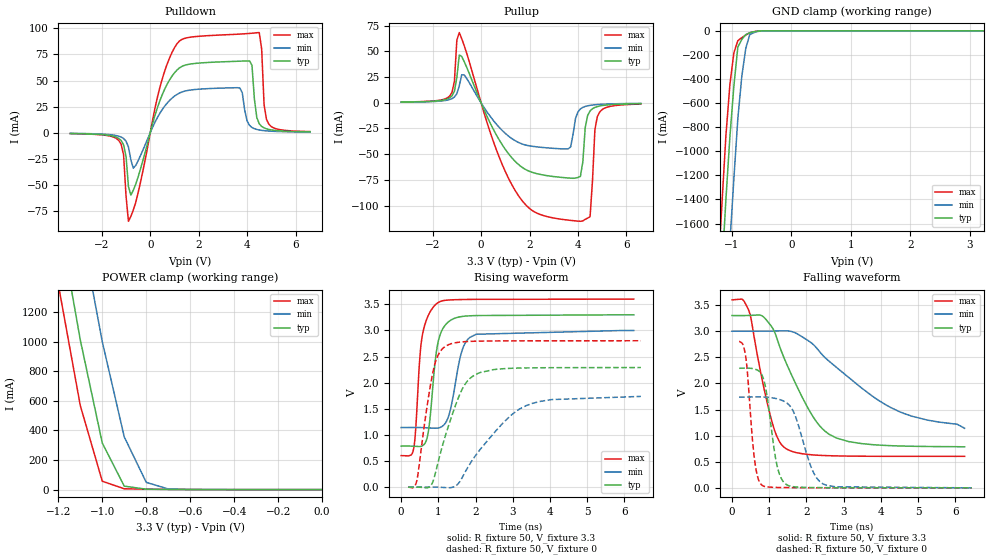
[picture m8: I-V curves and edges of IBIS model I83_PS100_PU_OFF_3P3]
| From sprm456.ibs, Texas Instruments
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|   Model Cell I83_PS100_PU_OFF_3P3
|IDG09_OUI83I83_PS100_PU_OFF_3P3
[Model]   I83_PS100_PU_OFF_3P3
Model_type   I/O
Polarity   Non-Inverting
Enable   Active-Low
Vinl =  0.8V
Vinh =  2V
Cref =  15pF
Rref =  100.00M
Vref =  0V
Vmeas =  1.65
C_comp   5.307p   5.123p   6.171p
[Model Spec]
Vinl   0.8V   0.8V   0.8V
Vinh   2V   2V   2V
[Temperature Range]   25   125   -40
[Voltage Range]   3.3   3   3.6
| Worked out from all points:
|   slope of the pulldown table from 0 to 0.495 V, typ, clamps not added: 13.6 ohm
|   slope of the pullup table from 0 to 0.495 V, typ, clamps not added: 19.6 ohm
|   GND clamp passes 1 mA (typ) near -0.52 V on its own axis
|   POWER clamp passes 1 mA (typ) near -0.67 V on its own axis
|   rising waveform, R_fixture 50, V_fixture 3.3: 20-80 % time 228ps typ, 309ps min, 198ps max; typ from 0.785 V to 3.3 V
|   rising waveform, R_fixture 50, V_fixture 0: 20-80 % time 625ps typ, 1.21ns min, 357ps max; typ from 0 V to 2.29 V
|   falling waveform, R_fixture 50, V_fixture 3.3: 20-80 % time 1.01ns typ, 2.01ns min, 530ps max; typ from 3.3 V to 0.785 V
|   falling waveform, R_fixture 50, V_fixture 0: 20-80 % time 276ps typ, 463ps min, 192ps max; typ from 2.29 V to 0 V
| Nom Voltages:
|   VDD=1.1, VDDS=3.3, VSS=0, VSSS=0
| Min Voltages:
|   VDD=1, VDDS=3, VSS=0, VSSS=0
| Max Voltages:
|   VDD=1.2, VDDS=3.6, VSS=0, VSSS=0
[POWER_clamp]
|   voltage   I(typ)   I(min)   I(max)
-3.3V     22.22A     22.93A     21.83A
-1.2V     1.856A     2.664A     1.387A
-1.167V   1.575A     2.376A     1.114A
-1.133V   1.294A     2.087A     841.3mA
-1.1V     1.013A     1.799A     568.3mA
-1.067V   780mA      1.533A     397.8mA
-1.033V   547.6mA    1.267A     227.3mA
-1V       315.1mA    1.001A     56.76mA
-900mV    23.42mA    356.5mA    5.611mA
-800mV    2.753mA    49.19mA    3.096mA
-700mV    1.202mA    4.273mA    1.5mA
0V        96.62pA    13.96nA    1.079pA
[Pulldown]
|   voltage   I(typ)   I(min)   I(max)
-3.3V     -826.1uA   -650.2uA   -901.2uA
-1.3V     -5.507mA   -3.361mA   -7.401mA
-1.1V     -11.64mA   -5.587mA   -21.3mA
-900mV    -51.57mA   -13.69mA   -84.93mA
-700mV    -55.24mA   -34.01mA   -74.16mA
1.1V      59.92mA    36.57mA    85.06mA
3.7V      68.51mA    42.82mA    94.48mA
4.1V      68.76mA    7.013mA    95.13mA
4.5V      8.571mA    2.593mA    95.94mA
4.7V      4.569mA    1.949mA    26.87mA
4.9V      3.077mA    1.558mA    8.021mA
6.6V      795.1uA    568.4uA    1.029mA
[Pullup]
|   voltage   I(typ)   I(min)   I(max)
-3.3V     663.7uA    556.1uA    740.7uA
-1.3V     4.799mA    3.15mA     6.471mA
-1.1V     11.28mA    5.644mA    21.14mA
-1V       24.69mA    8.858mA    61.1mA
-900mV    46.52mA    16.5mA     68.38mA
1.5V      -59.13mA   -38.08mA   -88.86mA
3.6V      -73.21mA   -44.75mA   -114.2mA
4.1V      -71.75mA   -5.995mA   -115.4mA
4.5V      -7.928mA   -2.493mA   -111mA
4.7V      -4.5mA     -1.913mA   -26.05mA
4.9V      -3.11mA    -1.549mA   -8.885mA
6.6V      -838.9uA   -584.8uA   -1.219mA
[GND_clamp]
|   voltage   I(typ)   I(min)   I(max)
-3.3V     -22.66A    -23.52A    -22.18A
-1.233V   -2.568A    -3.511A    -2.016A
-1.167V   -1.975A    -2.911A    -1.431A
-1.1V     -1.395A    -2.319A    -866.2mA
-1.033V   -879.1mA   -1.758A    -444.7mA
-966.7mV  -459.1mA   -1.228A    -183.3mA
-900mV    -135.1mA   -728.2mA   -81.84mA
-833.3mV  -71.1mA    -377.7mA   -56.6mA
-766.7mV  -31.45mA   -145.7mA   -34.78mA
-700mV    -16.16mA   -31.99mA   -16.38mA
-500mV    -447uA     -1.411mA   -156.1uA
3.233V    92.5pA     1.432uA    854.1fA
[Ramp]
| variable   typ   min   max
dV/dt_f  1.5152618/1.0114503n  1.1197432/2.0075258n  1.8066473/0.53161319n
dV/dt_r  1.3823108/0.62701275n  1.0497764/1.2136254n  1.6902155/0.35746376n
R_load = 50
[Rising Waveform]
R_fixture = 50
V_fixture = 3.3
V_fixture_min = 3
V_fixture_max = 3.6
|   time   V(typ)   V(min)   V(max)
0s        785.3mV    1.141V     603.3mV
334.7ps   783.6mV    1.142V     732.7mV
387.6ps   781.6mV    1.142V     1.077V
518.6ps   779.5mV    1.141V     2.621V
673ps     886.7mV    1.137V     3.189V
977.4ps   2.723V     1.131V     3.526V
1.267ns   3.162V     1.342V     3.583V
1.6ns     3.264V     2.526V     3.592V
1.845ns   3.281V     2.867V     3.594V
6.25ns    3.3V       3V         3.6V
[Rising Waveform]
R_fixture = 50
V_fixture = 0
V_fixture_min = 0
V_fixture_max = 0
|   time   V(typ)   V(min)   V(max)
192ps     0V         0V         0V
425.8ps   0V         0V         138.9mV
804.8ps   38.14mV    0V         2.02V
955.3ps   370.1mV    0V         2.466V
1.186ns   977.7mV    -8.865mV   2.695V
1.648ns   1.886V     193.7mV    2.782V
2.128ns   2.195V     725.6mV    2.796V
2.931ns   2.274V     1.362V     2.801V
3.518ns   2.284V     1.602V     2.802V
6.442ns   2.29V      1.737V     2.803V
[Falling Waveform]
R_fixture = 50
V_fixture = 3.3
V_fixture_min = 3
V_fixture_max = 3.6
|   time   V(typ)   V(min)   V(max)
0s        3.3V       3V         3.6V
278.2ps   3.299V     3V         3.609V
459.9ps   3.302V     3V         3.38V
1.054ns   3.098V     3.003V     1.32V
1.261ns   2.749V     3.005V     903.9mV
1.442ns   2.417V     3.007V     755.4mV
2.232ns   1.304V     2.711V     628.3mV
2.811ns   953mV      2.305V     612mV
4.275ns   807.7mV    1.535V     603.9mV
6.25ns    785.3mV    1.141V     603.3mV
[Falling Waveform]
R_fixture = 50
V_fixture = 0
V_fixture_min = 0
V_fixture_max = 0
|   time   V(typ)   V(min)   V(max)
192ps     2.29V      1.737V     2.803V
358.3ps   2.293V     1.738V     2.559V
605.9ps   2.275V     1.741V     542.5mV
821.6ps   2.135V     1.741V     42.62mV
1.206ns   443.2mV    1.706V     8.021mV
1.471ns   59.2mV     1.627V     5.14mV
1.711ns   17.34mV    1.357V     3.583mV
2.157ns   6.387mV    345mV      0V
2.438ns   4.48mV     78.8mV     0V
6.442ns   0V         0V         0V
